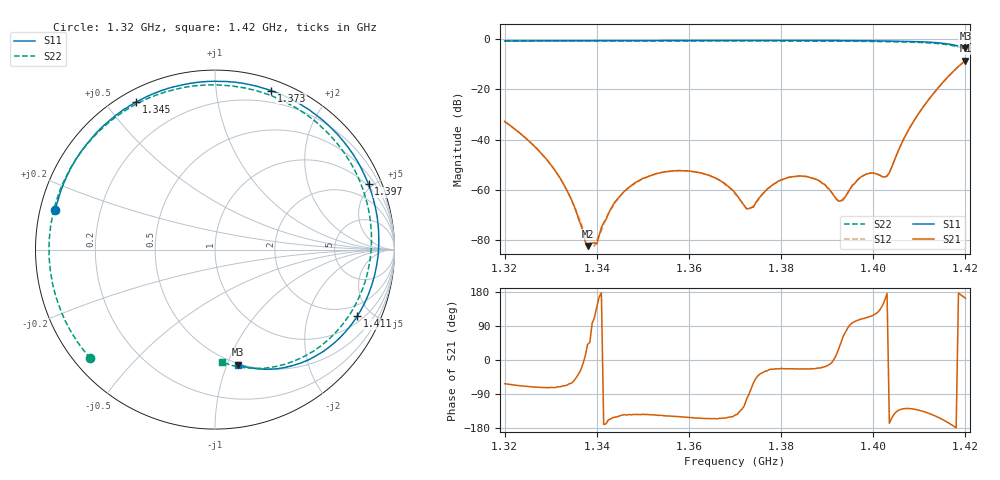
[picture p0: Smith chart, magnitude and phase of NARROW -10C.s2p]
!Agilent Technologies,E8363B,SG43030131,A.07.50.48
!Agilent E8363B: A.07.50.48
!Date: Friday, November 21, 2025 21:46:37
!Correction: S11(Full 2 Port(1,2))
!S21(Full 2 Port(1,2))
!S12(Full 2 Port(1,2))
!S22(Full 2 Port(1,2))
!S2P File: Measurements: S11, S21, S12, S22:
# Hz S  dB  R 50
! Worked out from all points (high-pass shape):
!   201 points, 1.32 GHz to 1.42 GHz, reference 50 ohm
!   highest |S21| = -8.55 dB at 1.42 GHz (marker M1); lowest = -82.4 dB at 1.338 GHz (marker M2)
!   |S21| within 3 dB of the highest: 1.418113 GHz to end of sweep
!   lowest |S11| = -3.7 dB at 1.42 GHz (marker M3), VSWR 4.77, Z = 24.5 - j54.7 ohm
!   |S11| at or under -10 dB: nowhere
!   |S22| runs from -4.1 to -0.7 dB; largest |S21 - S12| = 0.00036
!   S11 on the Smith chart (normalised r, x): 1.32 GHz: 0.04, +0.12; 1.345 GHz: 0.05, +0.60; 1.373 GHz: 0.09, +1.41; 1.397 GHz: 0.89, +4.75; 1.411 GHz: 1.29, -4.11; 1.42 GHz: 0.49, -1.09
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1.32e9  -0.76 166.1  -32.80 -62.6  -32.79 -62.7  -0.71 -138.9
1.3305e9  -0.68 144.0  -51.18 -72.7  -51.21 -72.3  -0.68 -161.0
1.3345e9  -0.66 136.3  -63.97 -61.3  -63.93 -59.2  -0.68 -169.0
1.337e9  -0.64 131.7  -76.62 -10.1  -75.59 -10.1  -0.68 -174.1
1.3375e9  -0.64 130.8  -80.67 10.6  -80.74 -19.2  -0.68 -175.1
1.338e9  -0.64 129.8  -82.38 40.7  -82.21 29.3  -0.68 -176.1
1.34e9  -0.63 126.1  -81.68 139.9  -79.89 132.7  -0.68 179.9
1.3445e9  -0.61 118.2  -63.64 -149.7  -64.00 -151.2  -0.68 170.9
1.3485e9  -0.59 111.2  -57.00 -143.8  -57.09 -143.1  -0.68 162.9
1.3535e9  -0.58 102.8  -53.34 -146.2  -53.37 -145.3  -0.69 152.8
1.363e9  -0.55 86.8  -53.53 -154.1  -53.50 -154.5  -0.70 133.1
1.37e9  -0.54 74.9  -61.31 -145.5  -61.78 -146.0  -0.71 117.9
1.3725e9  -0.54 70.6  -67.59 -103.5  -67.64 -108.0  -0.72 112.3
1.3795e9  -0.55 58.2  -56.47 -23.7  -56.63 -23.1  -0.74 95.8
1.387e9  -0.56 43.8  -55.47 -23.4  -55.64 -22.9  -0.77 76.3
1.3925e9  -0.59 32.3  -64.55 29.2  -64.59 27.9  -0.82 60.4
1.3965e9  -0.63 23.0  -56.30 104.2  -56.25 104.7  -0.87 47.5
1.4035e9  -0.77 4.2  -53.22 -167.0  -53.07 -167.6  -1.02 21.4
1.407e9  -0.89 -7.2  -38.41 -128.1  -38.42 -128.1  -1.15 5.8
1.4115e9  -1.16 -25.1  -25.38 -138.2  -25.38 -138.2  -1.46 -18.4
1.4165e9  -2.01 -52.6  -14.50 -167.2  -14.50 -167.2  -2.35 -54.0
1.42e9  -3.70 -78.8  -8.55 162.9  -8.55 162.9  -4.05 -86.6
